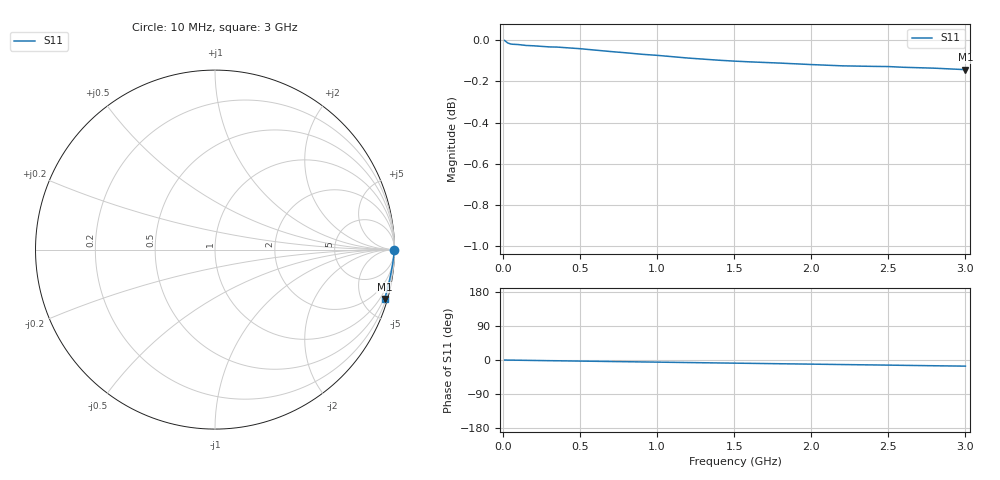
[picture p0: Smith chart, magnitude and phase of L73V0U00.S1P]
! SIEMENS Small Signal Semiconductors
! BAR14-1
! Si PIN Diode in SOT23
! VR = 3 V
! S-Parameters:  July  1992
# GHz  S  MA  R  50
!  f  S11
! GHz  MAG  ANG
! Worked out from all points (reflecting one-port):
!   31 points, 10 MHz to 3 GHz, reference 50 ohm
!   lowest |S11| = -0.1 dB at 3 GHz (marker M1), VSWR 121.70, Z = 20.6 - j350 ohm
!   phase of S11 starts at -0 deg and turns -16 deg over the sweep
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0.01  0.9999 -0.1
0.03  0.9985 -0.3
0.05  0.9979 -0.4
0.06  0.9978 -0.4
0.1  0.9976 -0.6
0.15  0.9971 -0.9
0.2  0.9969 -1.2
0.3  0.9963 -1.8
0.35  0.9962 -2.0
0.4  0.9959 -2.3
0.5  0.9953 -2.9
0.6  0.9945 -3.4
0.7  0.9937 -4.0
0.8  0.993 -4.5
0.9  0.9922 -5.1
1  0.9916 -5.6
1.2  0.9901 -6.7
1.4  0.9889 -7.8
1.5  0.9884 -8.3
1.6  0.988 -8.8
1.8  0.9873 -9.9
2  0.9865 -10.9
2.2  0.9858 -12.0
2.4  0.9855 -13.0
2.5  0.9854 -13.5
2.6  0.985 -14.1
2.8  0.9845 -15.2
3  0.9837 -16.2
